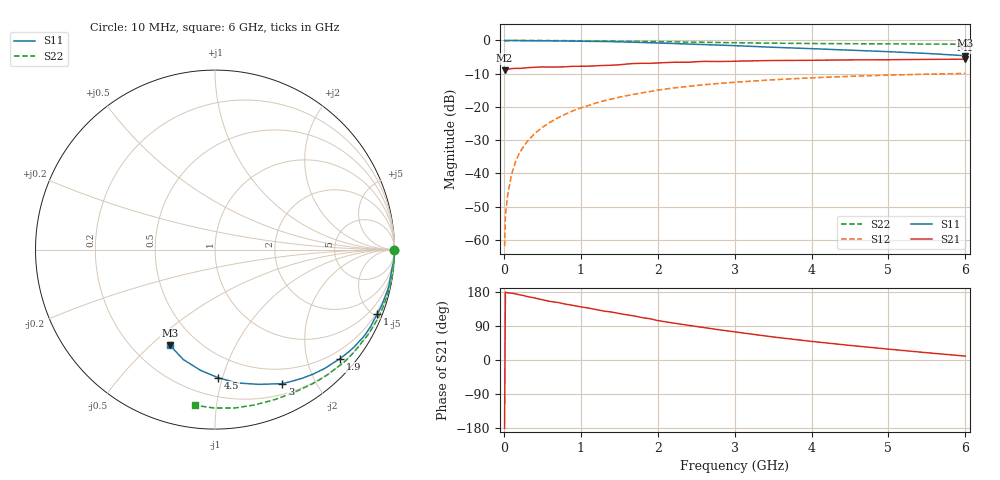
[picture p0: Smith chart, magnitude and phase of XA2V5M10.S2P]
! SIEMENS Discrete & RF Semiconductors
! BFY180
! Si NPN RF Bipolar Junction Transistor in MICRO-X
! VCE = 2.5 V  IC = 0.1 mA
! Common Emitter S-Parameters:  May  1997
# GHz  S  MA  R  50
!  f  S11  S21  S12  S22
! GHz  MAG  ANG  MAG  ANG  MAG  ANG  MAG  ANG
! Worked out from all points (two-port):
!   36 points, 10 MHz to 6 GHz, reference 50 ohm
!   highest |S21| = -5.63 dB at 6 GHz (marker M1); lowest = -9.0 dB at 10 MHz (marker M2)
!   |S21| within 3 dB of the highest: 52.15 MHz to end of sweep
!   lowest |S11| = -4.6 dB at 6 GHz (marker M3), VSWR 3.86, Z = 17.7 - j28.8 ohm
!   |S11| at or under -10 dB: nowhere
!   |S22| runs from -1.2 to 0.0 dB; largest |S21 - S12| = 0.4
!   S11 on the Smith chart (normalised r, x): 10 MHz: open; 1 GHz: 0.38, -5.22; 1.9 GHz: 0.32, -2.63; 3 GHz: 0.32, -1.58; 4.5 GHz: 0.33, -0.97; 6 GHz: 0.35, -0.58
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0.01  0.9958 -0.2  0.356 -179.8  0.0008 88.6  0.9992 -0.1
0.02  0.9848 -0.3  0.361 179.2  0.0023 94.0  0.9999 -0.3
0.05  0.9922 -0.8  0.37 177.2  0.0047 81.8  0.9991 -0.9
0.1  0.9996 -2.2  0.376 176.3  0.0096 88.1  0.9993 -1.9
0.15  0.9979 -3.2  0.381 174.6  0.0147 88.0  1 -2.8
0.2  0.9966 -4.3  0.38 172.1  0.0199 86.3  0.999 -3.8
0.3  0.9913 -6.4  0.388 167.5  0.0297 84.0  0.9981 -5.7
0.4  0.9899 -8.4  0.395 163.8  0.0396 82.4  0.9987 -7.5
0.5  0.9894 -11.1  0.399 158.9  0.0492 80.2  0.9972 -9.5
0.7  0.9836 -15.3  0.399 151.9  0.0681 76.0  0.9951 -13.3
1  0.9736 -21.6  0.409 140.2  0.0965 69.9  0.9893 -19.1
1.1  0.9687 -23.8  0.41 137.1  0.105 67.9  0.9877 -20.8
1.5  0.9524 -32.4  0.43 122.7  0.1399 59.9  0.977 -28.4
1.9  0.9239 -41.2  0.453 108.9  0.1704 52.1  0.9624 -35.6
2.2  0.9008 -47.4  0.47 97.6  0.1923 46.4  0.9552 -41.0
2.6  0.8671 -55.6  0.485 85.6  0.2155 39.4  0.9388 -47.5
3  0.8358 -63.3  0.487 74.3  0.2347 32.5  0.9243 -53.9
3.5  0.7896 -72.0  0.499 60.8  0.256 25.2  0.9097 -61.2
4  0.7525 -80.7  0.503 49.1  0.2738 18.1  0.8995 -68.4
4.5  0.7143 -88.5  0.51 38.5  0.2884 11.4  0.8934 -75.6
5.5  0.6375 -106.1  0.519 19.2  0.3109 -1.7  0.8826 -90.3
6  0.5889 -115.3  0.523 10.3  0.3188 -8.3  0.8745 -97.5
